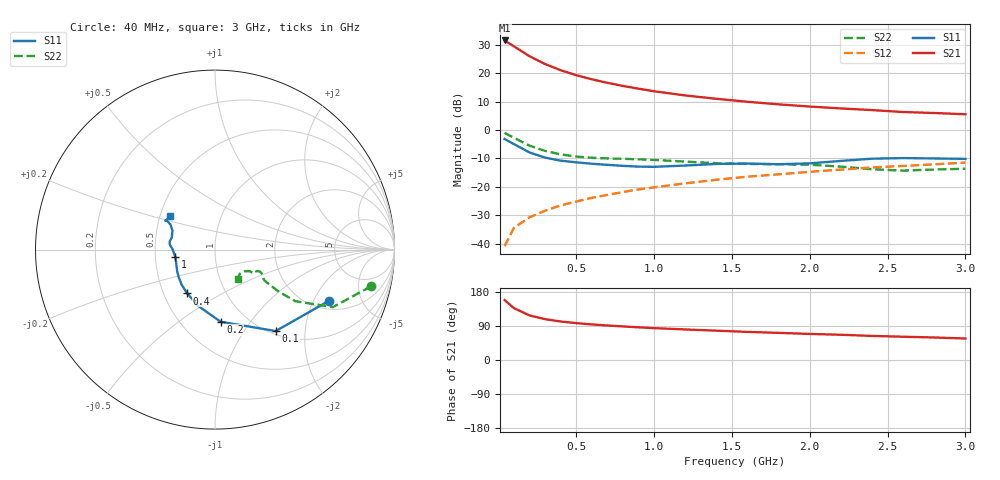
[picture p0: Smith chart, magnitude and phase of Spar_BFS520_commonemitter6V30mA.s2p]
! Filename:  BFS520L.S2P  Version:  4.0
! NXP part #: BFS520  Date: Jun 1994
! Bias condition: Vce=6V, Ic=30mA
#  MHz  S  MA  R  50
! Freq  S11  S21  S12  S22  !GUM [dB]
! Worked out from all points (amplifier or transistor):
!   21 points, 40 MHz to 3 GHz, reference 50 ohm
!   highest |S21| = 31.6 dB at 40 MHz (marker M1)
!   |S21| within 3 dB of that: start of sweep to 126.7 MHz
!   unconditionally stable (mu >= 1): 577 MHz to end of sweep
!   at 300 MHz: K = 0.84, MSG = 25.8 dB, |S12| = -28.4 dB
!   at 1 GHz: K = 1.08, MAG = 15.2 dB, |S12| = -20.2 dB
!   at 3 GHz: K = 1.05, MAG = 7.1 dB, |S12| = -11.5 dB
!   S11 on the Smith chart (normalised r, x): 40 MHz: 2.41, -2.67; 100 MHz: 1.06, -1.41; 200 MHz: 0.76, -0.73; 400 MHz: 0.66, -0.35; 1 GHz: 0.64, -0.05; 3 GHz: 0.57, +0.23
40  0.697 -24.1  37.92 158.2  0.009 78.9  0.892 -13.3
100  0.566 -53.3  29.89 136.8  0.019 68.6  0.731 -26.0
200  0.403 -85.6  20 117.6  0.029 64.4  0.532 -32.7
300  0.327 -106.7  14.57 107.8  0.038 65.6  0.429 -33.4
400  0.289 -122.4  11.35 101.6  0.047 67.7  0.373 -32.9
500  0.27 -133.3  9.276 97.3  0.055 69.4  0.341 -32.4
600  0.255 -141.9  7.845 93.9  0.064 70.4  0.325 -31.9
700  0.244 -149.4  6.799 91.1  0.072 71.6  0.316 -31.2
800  0.234 -156.2  5.989 88.6  0.081 72.4  0.312 -30.1
900  0.227 -162.7  5.357 86.2  0.09 72.8  0.305 -28.9
1000  0.225 -169.8  4.834 84.1  0.098 73.3  0.298 -27.6
1200  0.237 179.3  4.075 80.6  0.115 73.5  0.278 -25.9
1400  0.253 173.8  3.557 77.4  0.133 74.0  0.261 -27.2
1600  0.257 170.2  3.151 74.2  0.151 73.3  0.253 -30.9
1800  0.25 164.5  2.838 71.6  0.166 73.3  0.25 -32.1
2000  0.259 156.0  2.596 68.8  0.184 72.9  0.245 -31.7
2200  0.286 150.5  2.406 66.6  0.201 72.7  0.227 -31.9
2400  0.313 148.9  2.249 63.5  0.22 72.1  0.204 -36.2
2600  0.321 149.8  2.08 61.4  0.233 71.1  0.193 -44.3
2800  0.316 148.3  1.998 59.4  0.249 71.0  0.202 -50.1
3000  0.311 143.0  1.899 56.7  0.267 70.2  0.208 -51.9
